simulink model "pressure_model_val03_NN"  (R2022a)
settings: Solver=VariableStepAuto  StartTime=0.0  StopTime=tfin  RelTol=1e-3
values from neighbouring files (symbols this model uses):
  Ts = 5    [sisopres.m]
undefined symbols (not defined in the file or in its folder): magnitude
libraries: neural x16

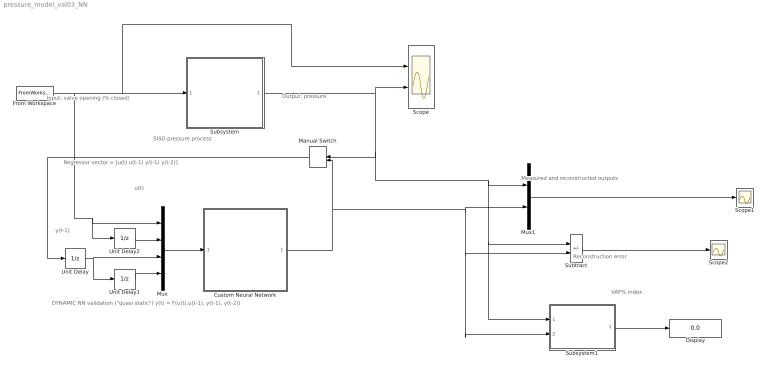
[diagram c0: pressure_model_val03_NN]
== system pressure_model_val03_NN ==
  note: VAF% index
  note: Measured and reconstructed outputs
  note: Regressor vector = [u(t) u(t-1) y(t-1) y(t-2)]
  note: y(t-1)
  note: u(t)
  note: DYNAMIC NN validation ("quasi static") y(t) = F(u(t),u(t-1), y(t-1), y(t-2))
  note: Output: pressure
  note: Input: valve opening (% closed)
  note: SISO pressure process
  note: Reconstruction error
  Custom Neural Network : Subsystem
      mask help: Custom Neural Network
  Display : Display
  From Workspace : FromWorkspace  VariableName=[tsim U]  SampleTime=Ts
  Manual Switch : ManualSwitch  CurrentSetting=0
  Mux : Mux
  Mux1 : Mux  Inputs=2
  Scope : Scope  NumInputPorts=2
  Scope1 : Scope
  Scope2 : Scope
  Subsystem : Subsystem
  Subsystem1 : Subsystem
  Subtract : Sum  Inputs=+-
  Unit Delay : UnitDelay  SampleTime=Ts  HasFrameUpgradeWarning=on
  Unit Delay1 : UnitDelay  SampleTime=Ts  HasFrameUpgradeWarning=on
  Unit Delay2 : UnitDelay  SampleTime=Ts  HasFrameUpgradeWarning=on
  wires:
  From Workspace/1 -> Scope/1, Subsystem/1(u), Unit Delay2/1, Mux/1
  Mux/1 -> Custom Neural Network/1(Input)
  Subsystem1/1(VAF%) -> Display/1
  Subtract/1 -> Scope2/1
  Subsystem/1(y) -> Manual Switch/1, Subsystem1/1(y_mis), Subtract/1, Mux1/1, Scope/2
  Custom Neural Network/1(Output) -> Manual Switch/2, Subsystem1/2(y_prev), Subtract/2, Mux1/2
  Mux1/1 -> Scope1/1
  Manual Switch/1 -> Unit Delay/1
  Unit Delay2/1 -> Mux/2
  Unit Delay1/1 -> Mux/4
  Unit Delay/1 -> Unit Delay1/1, Mux/3

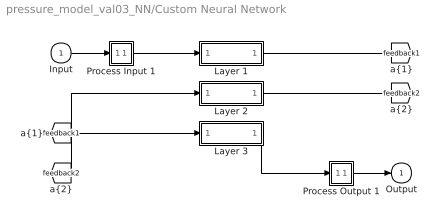
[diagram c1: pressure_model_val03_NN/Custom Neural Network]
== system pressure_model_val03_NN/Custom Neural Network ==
  Input : Inport  PortDimensions=4  SampleTime=5
  Layer 1 : Subsystem
  Layer 2 : Subsystem
  Layer 3 : Subsystem
  Process Input 1 : Subsystem
  Process Output 1 : Subsystem
  Output : Outport  InitialOutput=0
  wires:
  Input/1 -> Process Input 1/1(x)
  Process Output 1/1(y) -> Output/1
  Process Input 1/1(p) -> Layer 1/1("p{1}")
  Layer 1/1("a{1}") -> [feedback1]
  [feedback1] -> Layer 2/1("a{1} ")
  Layer 2/1("a{2}") -> [feedback2]
  [feedback2] -> Layer 3/1("a{2} ")
  Layer 3/1("a{3}") -> Process Output 1/1(a)

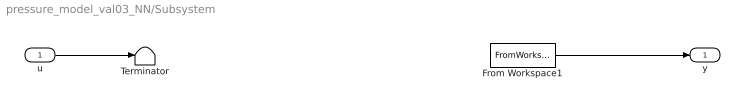
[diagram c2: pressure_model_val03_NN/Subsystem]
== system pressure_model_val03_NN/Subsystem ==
  u : Inport
  From Workspace1 : FromWorkspace  VariableName=[tsim Y]  SampleTime=Ts
  Terminator : Terminator
  y : Outport
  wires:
  From Workspace1/1 -> y/1
  u/1 -> Terminator/1

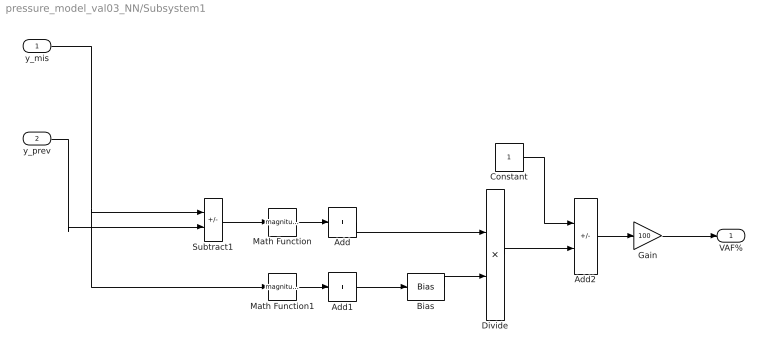
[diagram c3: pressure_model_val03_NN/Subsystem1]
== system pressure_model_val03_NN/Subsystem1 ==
  y_mis : Inport
  y_prev : Inport  Port=2
  Add : Sum  Inputs=+
  Add1 : Sum  Inputs=+
  Add2 : Sum  Inputs=+-
  Bias : Bias  Bias=1e-7
  Constant : Constant
  Divide : Product  Inputs=*/
  Gain : Gain  Gain=100
  Math Function : Math  Operator=magnitude^2
  Math Function1 : Math  Operator=magnitude^2
  Subtract1 : Sum  Inputs=+-
  VAF% : Outport
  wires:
  Add2/1 -> Gain/1
  Math Function/1 -> Add/1
  Bias/1 -> Divide/2
  y_mis/1 -> Math Function1/1, Subtract1/1
  Add1/1 -> Bias/1
  Math Function1/1 -> Add1/1
  Subtract1/1 -> Math Function/1
  Constant/1 -> Add2/1
  Divide/1 -> Add2/2
  Add/1 -> Divide/1
  y_prev/1 -> Subtract1/2
  Gain/1 -> VAF%/1

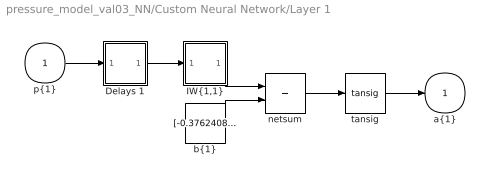
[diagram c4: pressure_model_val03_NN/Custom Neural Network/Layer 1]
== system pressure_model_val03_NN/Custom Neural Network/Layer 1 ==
  "p{1}" : Inport  PortDimensions=4  SampleTime=5
  Delays 1 : Subsystem
  "IW{1,1}" : Subsystem
  "b{1}" : Constant  Value=[-0.37624088256944310248996998780057765543460845947265625;-2.723542772668203770791706119780428707599639892578125;1.19986620356411943788543794653378427028656005859375;0.89635617322992333644293694305815733969211578369140625]
  netsum : Sum  Inputs=2  InputSameDT=on  SaturateOnIntegerOverflow=on
  tansig : neural/Transfer Functions/tansig
  "a{1}" : Outport  InitialOutput=[0;0;0;0]
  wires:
  "p{1}"/1 -> Delays 1/1("p{1}")
  Delays 1/1("pd{1,1}") -> "IW{1,1}"/1("pd{1,1}")
  "IW{1,1}"/1("iz{1,1}") -> netsum/1
  "b{1}"/1 -> netsum/2
  netsum/1 -> tansig/1
  tansig/1 -> "a{1}"/1

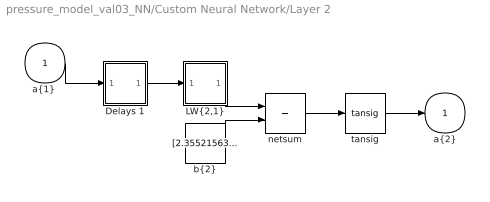
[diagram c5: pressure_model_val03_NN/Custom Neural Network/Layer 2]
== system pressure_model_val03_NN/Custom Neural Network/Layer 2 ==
  "a{1} " : Inport  PortDimensions=4  SampleTime=5
  Delays 1 : Subsystem
  "LW{2,1}" : Subsystem
  "b{2}" : Constant  Value=[2.355215638657059518124015085049904882907867431640625;-1.7519309409369296925973458201042376458644866943359375;-1.0258607299776312249406373666715808212757110595703125;0.2387798302893175128591707334635430015623569488525390625;-0.392042171458255150895411134115420281887054443359375;-0.8838088800359706898035483391140587627887725830078125;1.6005734331728138641892655869014561176300048828125;2.3455158238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
  netsum : Sum  Inputs=2  InputSameDT=on  SaturateOnIntegerOverflow=on
  tansig : neural/Transfer Functions/tansig
  "a{2}" : Outport  InitialOutput=[0;0;0;0;0;0;0;0]
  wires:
  "a{1} "/1 -> Delays 1/1("p{2}")
  Delays 1/1("pd{2,1}") -> "LW{2,1}"/1("ad{2,1}")
  "LW{2,1}"/1("lz{2,1}") -> netsum/1
  "b{2}"/1 -> netsum/2
  netsum/1 -> tansig/1
  tansig/1 -> "a{2}"/1

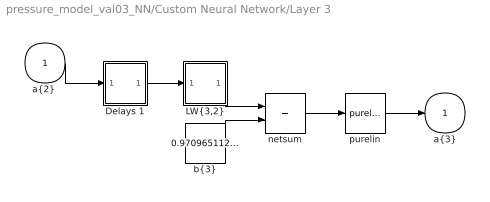
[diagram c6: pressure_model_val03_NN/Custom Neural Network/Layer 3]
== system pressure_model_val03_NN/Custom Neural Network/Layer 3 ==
  "a{2} " : Inport  PortDimensions=8  SampleTime=5
  Delays 1 : Subsystem
  "LW{3,2}" : Subsystem
  "b{3}" : Constant  Value=0.97096511222878145730419419123791158199310302734375
  netsum : Sum  Inputs=2  InputSameDT=on  SaturateOnIntegerOverflow=on
  purelin : neural/Transfer Functions/purelin
  "a{3}" : Outport  InitialOutput=0
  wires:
  "a{2} "/1 -> Delays 1/1("p{3}")
  Delays 1/1("pd{3,2}") -> "LW{3,2}"/1("ad{3,2}")
  "LW{3,2}"/1("lz{3,2}") -> netsum/1
  "b{3}"/1 -> netsum/2
  netsum/1 -> purelin/1
  purelin/1 -> "a{3}"/1

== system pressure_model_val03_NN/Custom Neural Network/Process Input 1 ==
  x : Inport  PortDimensions=4  SampleTime=5
  p : Outport  PortDimensions=4  SampleTime=5
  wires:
  x/1 -> p/1

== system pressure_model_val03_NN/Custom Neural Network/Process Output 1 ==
  a : Inport  PortDimensions=1  SampleTime=5
  y : Outport  PortDimensions=1  SampleTime=5
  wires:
  a/1 -> y/1

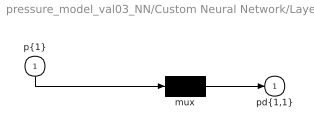
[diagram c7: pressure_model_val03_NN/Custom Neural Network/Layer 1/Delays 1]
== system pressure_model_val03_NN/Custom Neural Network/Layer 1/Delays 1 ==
  "p{1}" : Inport  PortDimensions=4  SampleTime=5
  mux : Mux  Inputs=1
  "pd{1,1}" : Outport
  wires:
  "p{1}"/1 -> mux/1
  mux/1 -> "pd{1,1}"/1

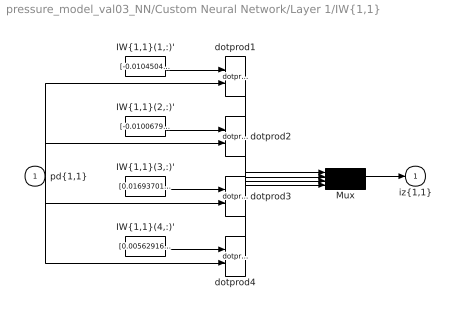
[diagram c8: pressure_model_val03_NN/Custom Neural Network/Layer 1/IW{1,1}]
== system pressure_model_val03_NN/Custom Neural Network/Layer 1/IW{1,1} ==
  "pd{1,1}" : Inport  PortDimensions=4  SampleTime=5
  "IW{1,1}(1,:)'" : Constant  Value=[-0.0104504249511474071876460101293560001067817211151123046875;-0.0586114319124515781300743810788844712078571319580078125;-1.4855167482781013177373097278177738189697265625;-0.59682697781708060613681254835682921111583709716796875]
  "IW{1,1}(2,:)'" : Constant  Value=[-0.01006793519306155119952261856042241561226546764373779296875;0.0284740882186545786469711316613029339350759983062744140625;-0.74209633344594083670386908124783076345920562744140625;1.243564621439840589545156035455875098705291748046875]
  "IW{1,1}(3,:)'" : Constant  Value=[0.016937016115608320709906564616176183335483074188232421875;-0.032707274748664132146824812252816627733409404754638671875;1.091337668899023949364845975651405751705169677734375;-1.425014074753556680974497794522903859615325927734375]
  "IW{1,1}(4,:)'" : Constant  Value=[0.00562916239460324076271380278058131807483732700347900390625;-0.01228883022140370671893006004893322824500501155853271484375;0.8759443045564114793677390480297617614269256591796875;-0.6050296561129251404764772814814932644367218017578125]
  Mux : Mux
  dotprod{1..4} (4 alike) : neural/Weight Functions/dotprod
  "iz{1,1}" : Outport
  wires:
  "IW{1,1}(1,:)'"/1 -> dotprod1/1
  "pd{1,1}"/1 -> dotprod1/2, dotprod2/2, dotprod3/2, dotprod4/2
  dotprod1/1 -> Mux/1
  "IW{1,1}(2,:)'"/1 -> dotprod2/1
  dotprod2/1 -> Mux/2
  "IW{1,1}(3,:)'"/1 -> dotprod3/1
  dotprod3/1 -> Mux/3
  "IW{1,1}(4,:)'"/1 -> dotprod4/1
  dotprod4/1 -> Mux/4
  Mux/1 -> "iz{1,1}"/1

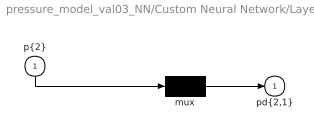
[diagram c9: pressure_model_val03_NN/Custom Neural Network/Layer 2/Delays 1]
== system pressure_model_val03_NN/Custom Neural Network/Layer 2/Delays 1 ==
  "p{2}" : Inport  PortDimensions=4  SampleTime=5
  mux : Mux  Inputs=1
  "pd{2,1}" : Outport
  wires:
  "p{2}"/1 -> mux/1
  mux/1 -> "pd{2,1}"/1

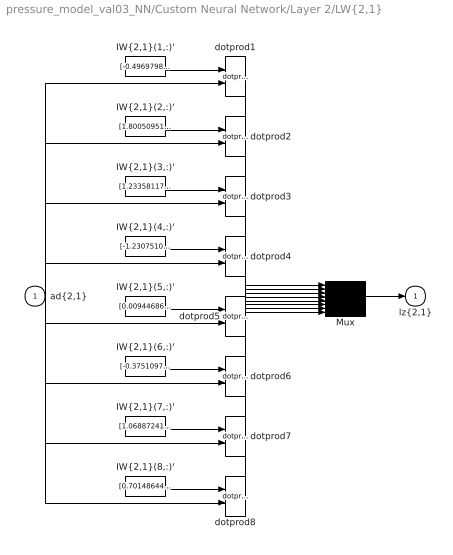
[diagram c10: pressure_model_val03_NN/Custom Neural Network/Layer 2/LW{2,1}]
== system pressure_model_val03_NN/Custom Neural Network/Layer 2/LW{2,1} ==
  "ad{2,1}" : Inport  PortDimensions=4  SampleTime=5
  "IW{2,1}(1,:)'" : Constant  Value=[-0.49697989088759653153459794339141808450222015380859375;1.066989485212505694988749382901005446910858154296875;-0.66813746734302181806697262800298631191253662109375;1.926800702024741074325220324681140482425689697265625]
  "IW{2,1}(2,:)'" : Constant  Value=[1.8005095111888598236049574552453123033046722412109375;-1.38504393491663702064897734089754521846771240234375;0.5093809459882925327889324762509204447269439697265625;0.239011349073253887009826712528592906892299652099609375]
  "IW{2,1}(3,:)'" : Constant  Value=[1.23358117412592349637634470127522945404052734375;0.7402368639665695138063483682344667613506317138671875;-1.1228520468435532198014925597817637026309967041015625;-1.5010352389646233195463764786836691200733184814453125]
  "IW{2,1}(4,:)'" : Constant  Value=[-1.2307510275709609981475978202070109546184539794921875;0.42785193173252034082310046869679354131221771240234375;1.1817360272182269032015256016165949404239654541015625;-1.51938918900727149008389460504986345767974853515625]
  "IW{2,1}(5,:)'" : Constant  Value=[0.00944686067957219155477588401481625624001026153564453125;-1.7404224169933784072128446496208198368549346923828125;-1.30156369820206574416943112737499177455902099609375;-1.3421597749836753354912843860802240669727325439453125]
  "IW{2,1}(6,:)'" : Constant  Value=[-0.37510972376741713585346360559924505650997161865234375;-1.70412568228449412544023289228789508342742919921875;-0.1004553927545751845773480681600631214678287506103515625;1.6647895019964493723563236926565878093242645263671875]
  "IW{2,1}(7,:)'" : Constant  Value=[1.0688724122413919559448913787491619586944580078125;0.0123569707163072826927585623479899368248879909515380859375;1.3806345116348042179055255473940633237361907958984375;-1.67822999949012086062793969176709651947021484375]
  "IW{2,1}(8,:)'" : Constant  Value=[0.7014864425395435088006479418254457414150238037109375;1.5061559997732907323353401807253248989582061767578125;1.31873299316718917140178746194578707218170166015625;1.03456862209281030828833536361344158649444580078125]
  Mux : Mux  Inputs=8
  dotprod{1..8} (8 alike) : neural/Weight Functions/dotprod
  "lz{2,1}" : Outport
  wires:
  "IW{2,1}(1,:)'"/1 -> dotprod1/1
  "ad{2,1}"/1 -> dotprod1/2, dotprod2/2, dotprod3/2, dotprod4/2, dotprod5/2, dotprod6/2, dotprod7/2, dotprod8/2
  dotprod1/1 -> Mux/1
  "IW{2,1}(2,:)'"/1 -> dotprod2/1
  dotprod2/1 -> Mux/2
  "IW{2,1}(3,:)'"/1 -> dotprod3/1
  dotprod3/1 -> Mux/3
  "IW{2,1}(4,:)'"/1 -> dotprod4/1
  dotprod4/1 -> Mux/4
  "IW{2,1}(5,:)'"/1 -> dotprod5/1
  dotprod5/1 -> Mux/5
  "IW{2,1}(6,:)'"/1 -> dotprod6/1
  dotprod6/1 -> Mux/6
  "IW{2,1}(7,:)'"/1 -> dotprod7/1
  dotprod7/1 -> Mux/7
  "IW{2,1}(8,:)'"/1 -> dotprod8/1
  dotprod8/1 -> Mux/8
  Mux/1 -> "lz{2,1}"/1

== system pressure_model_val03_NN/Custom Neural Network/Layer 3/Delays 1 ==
  "p{3}" : Inport  PortDimensions=8  SampleTime=5
  mux : Mux  Inputs=1
  "pd{3,2}" : Outport
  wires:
  "p{3}"/1 -> mux/1
  mux/1 -> "pd{3,2}"/1

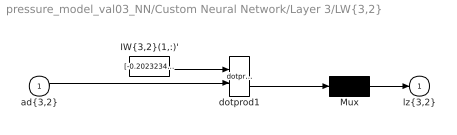
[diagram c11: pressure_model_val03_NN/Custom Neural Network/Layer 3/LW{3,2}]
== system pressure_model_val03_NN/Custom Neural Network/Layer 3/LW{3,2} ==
  "ad{3,2}" : Inport  PortDimensions=8  SampleTime=5
  "IW{3,2}(1,:)'" : Constant  Value=[-0.2023234024203163505806202238090918399393558502197265625;0.454934494356577123763685222002095542848110198974609375;-0.5929874606830640715315894340164959430694580078125;-0.856906904939803037990486700437031686305999755859375;-0.95945197267809223529155815413105301558971405029296875;0.1278505795425858571068289393224404193460941314697265625;-0.56226052517134983421698279926204122602939605712890625;-0.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
  Mux : Mux  Inputs=1
  dotprod1 : neural/Weight Functions/dotprod
  "lz{3,2}" : Outport
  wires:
  "IW{3,2}(1,:)'"/1 -> dotprod1/1
  "ad{3,2}"/1 -> dotprod1/2
  dotprod1/1 -> Mux/1
  Mux/1 -> "lz{3,2}"/1
